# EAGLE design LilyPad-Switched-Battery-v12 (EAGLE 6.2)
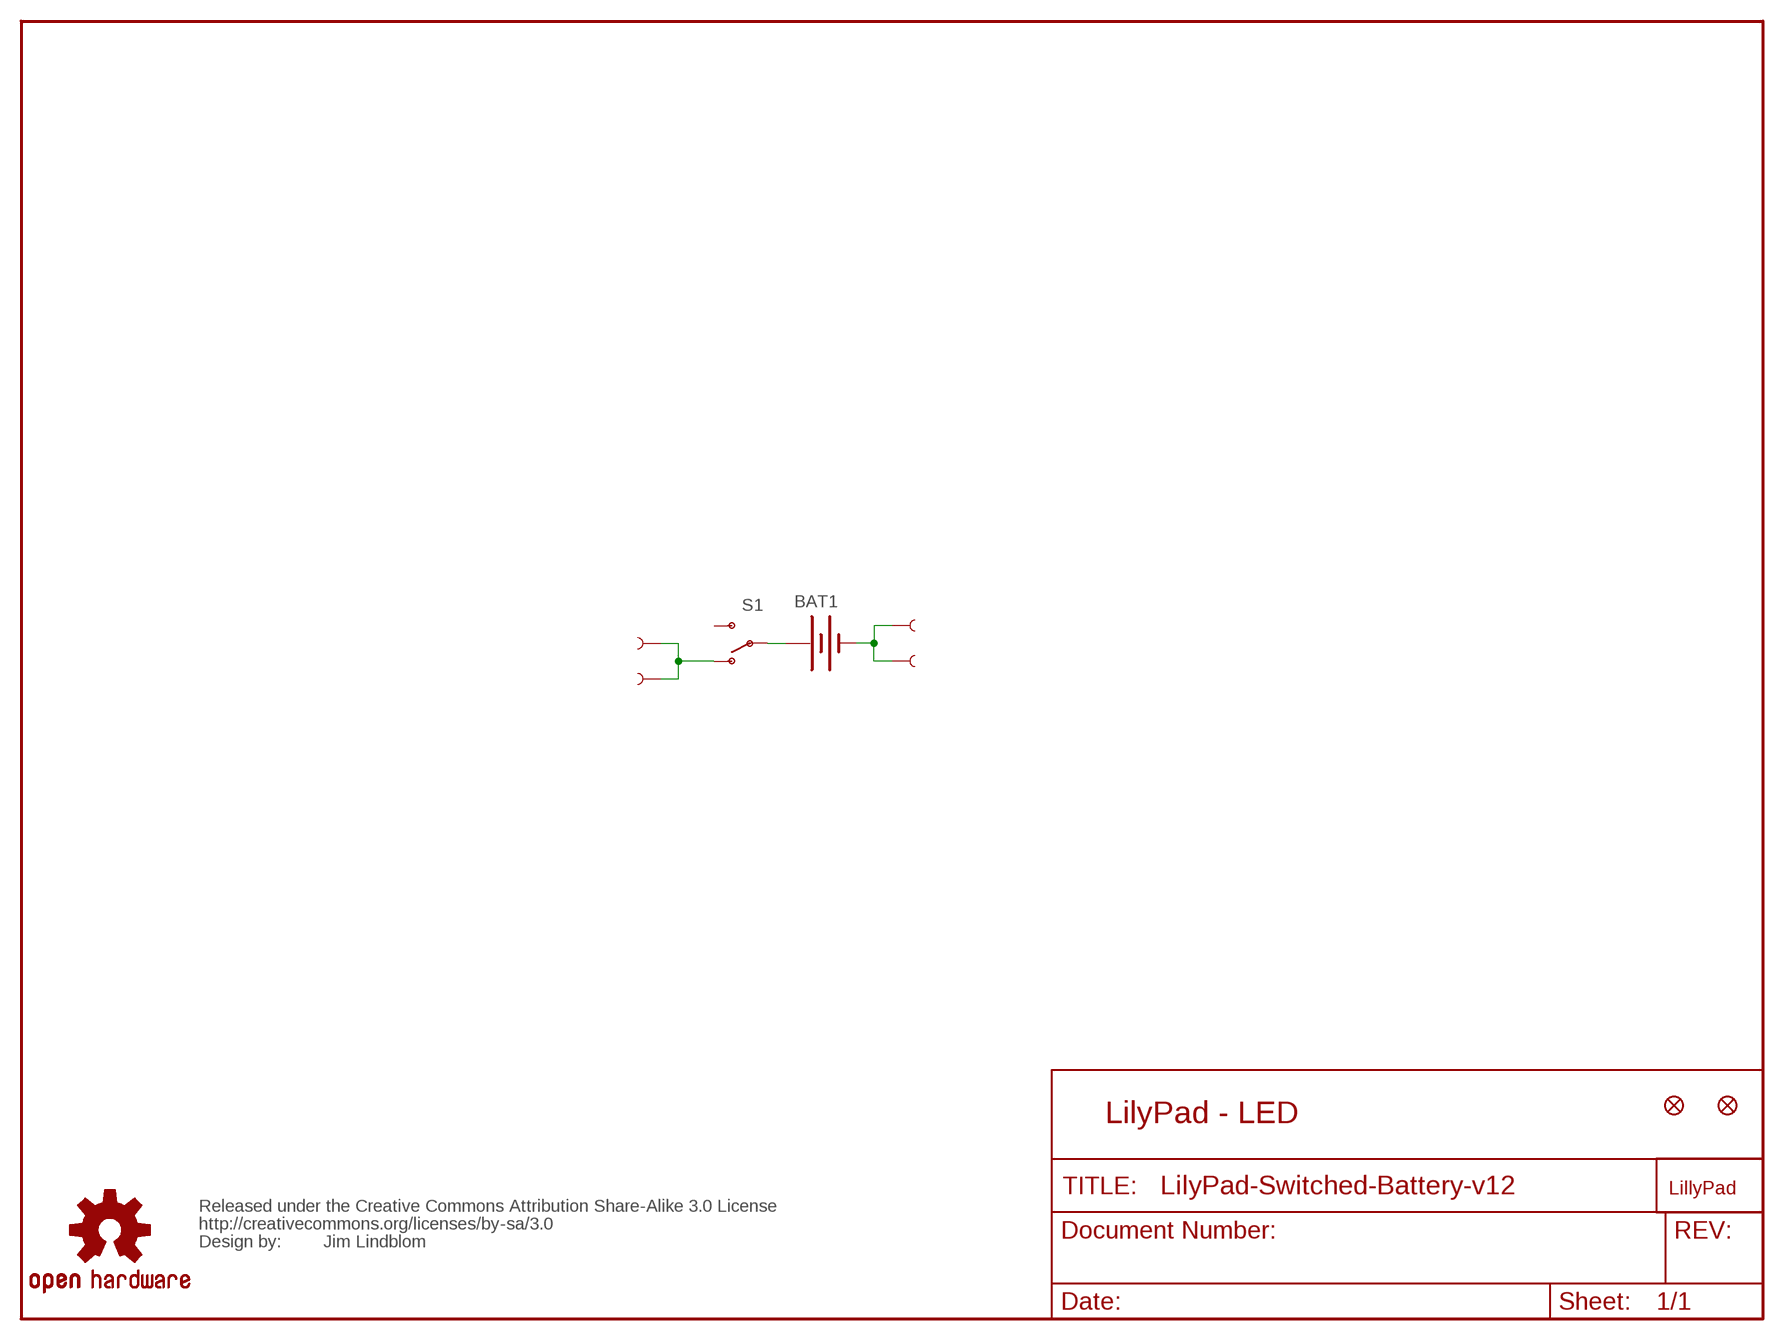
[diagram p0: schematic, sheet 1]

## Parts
BAT1  BATTERY20MM_4LEGS  [BATTCON_20MM_4LEGS]
JP1  FIDUCIALUFIDUCIAL  [MICRO-FIDUCIAL]
JP2  FIDUCIALUFIDUCIAL  [MICRO-FIDUCIAL]
S1  SWITCH-SPSTSMD  [AYZ0202]
U$1  SEWTAP6  [PETAL-SMALL-2SIDE]
U$2  SEWTAP6  [PETAL-SMALL-2SIDE]
U$3  SEWTAP6  [PETAL-SMALL-2SIDE]
U$4  SEWTAP6  [PETAL-SMALL-2SIDE]
U$5  LOGO-LPLP  [LOGO-LILYPAD]
U$7  OSHW-LOGOS  [OSHW-LOGO-S]
U$8  CREATIVE_COMMONS  [CREATIVE_COMMONS]

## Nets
N$1: S1.1(O) U$2.1 U$4.1
N$2: BAT1.2(-) U$1.1 U$3.1
N$3: BAT1.1(+) BAT1.3(+) BAT1.P$1(+) BAT1.P$2(+) S1.2(P)
Unconnected: S1.3(S)

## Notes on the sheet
- LilyPad - LED
- Jim Lindblom

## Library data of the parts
BAT1 = SparkFun-Electromechanical:BATTERY: Battery Holders
JP1 JP2 = SparkFun:FIDUCIAL: Fiducial Alignment Points
S1 = SparkFun:SWITCH-SPST: SPST Switch Simple slide switch. Spark Fun Electronics SKU : COM-00102
U$1-U$4 = LilyPad-Wearables:SEWTAP
U$5 = LilyPad-Wearables:LOGO-LP
U$7 = SparkFun-Aesthetics:OSHW-LOGO: Open Source Hardware Logo This logo indicates the piece of hardware it is found on incorporates a OSHW license and/or adheres to the definition of open source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
U$8 = SparkFun-Aesthetics:CREATIVE_COMMONS: Creative Commons License summary

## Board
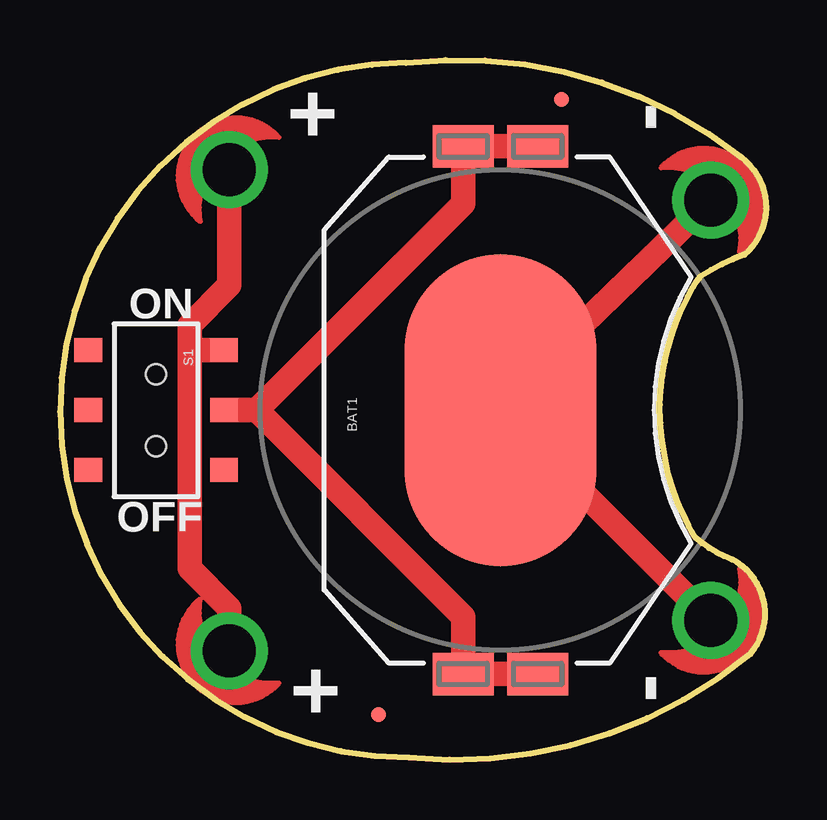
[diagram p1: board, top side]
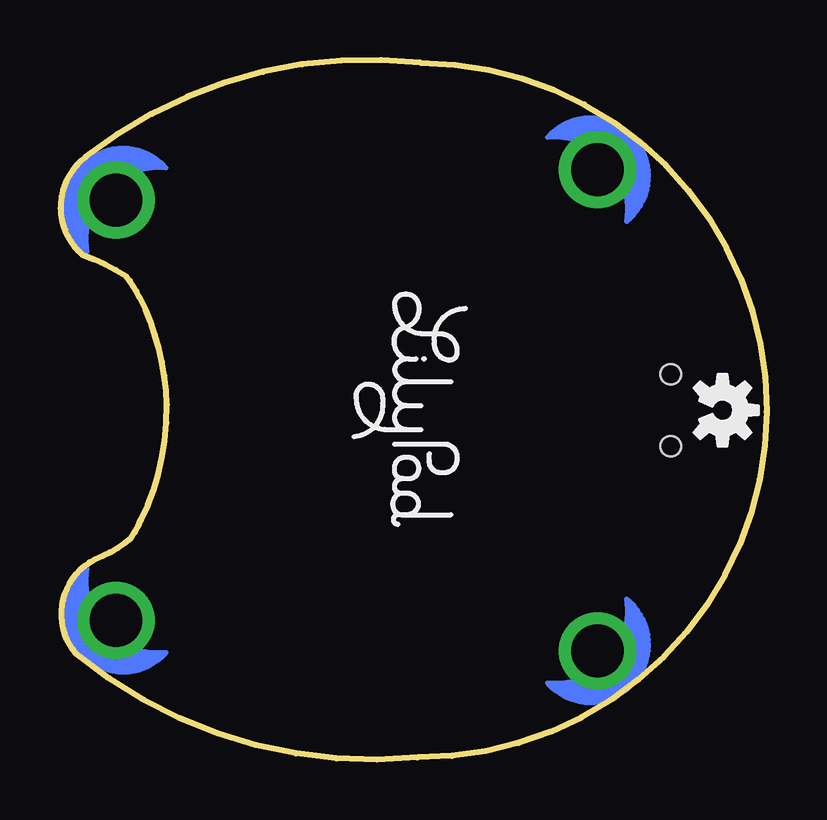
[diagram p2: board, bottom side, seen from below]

Size 29.42 x 29.17 mm. Coordinates in mm from the lower left corner, seen from the top.
Outline: 14.54,0.09 arc45 28.77,4.41 arc103 28,8.35 arc-20 26.48,9.25 arc-11 26.07,9.99 arc-17 25.21,12.55 arc-11 24.99,14.8 arc-13 25.34,17.17 arc-9 25.88,18.76 26.15,19.29 arc-14 26.7,20.16 arc-13 28.51,21.05 arc102 28.38,25.11 arc45 14.41,29.05 arc180 14.54,0.09
Copper layers (1*16): Top 0.035mm / dielectric 1.5mm / Bottom 0.035mm
Design rules: minimum track width 8mil, minimum drill 20mil, track to track 8mil, track to pad 8mil, pad to pad 8mil, via to via 8mil, smd to smd 8mil, copper to edge 8mil, drill to drill 8mil, minimum pad ring 12mil, minimum via ring 10mil, stop-mask expansion 4mil, vias tented up to drill 20mil, thermal gap 10mil

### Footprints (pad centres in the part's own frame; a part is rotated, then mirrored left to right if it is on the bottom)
BATTCON_20MM_4LEGS = smd 1.778 x 2.54: 1 -11,1.55; 3 11,1.55; P$1 -11,-1.55; P$2 11,-1.55 | smd 13 x 8: 2 0,0
MICRO-FIDUCIAL = smd 0.635 x 0.635: 1 0,0
AYZ0202 = smd 1 x 1.15: 1 -2.5,2.825; 2 0,2.825; 3 2.5,2.825; 4 -2.5,-2.825; 5 0,-2.825; 6 2.5,-2.825 | hole 0.85: 1.5,0; -1.5,0
PETAL-SMALL-2SIDE = drill 2.2: 1 0,0

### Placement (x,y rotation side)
BAT1  18.35,14.57 90 top
JP1  13.27,1.87 0 top
JP2  20.89,27.52 0 top
S1  4,14.57 270 top
U$1  27.11,5.81 47 top
U$2  7.05,4.54 313 top
U$3  27.11,23.33 133 top
U$4  7.05,24.6 227 top
U$5  14.54,14.57 270 bottom
U$7  1.84,14.57 270 bottom
U$8  not placed on the board

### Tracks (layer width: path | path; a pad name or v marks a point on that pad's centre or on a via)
N$1
  Top 1.016: U$4.1 7.05,19.78 5.4,18.13 5.4,17.11 | 5.4,17.11 5.4,7.97 7.05,6.32 U$2.1 | S1.1 5.44,17.07 5.4,17.11
N$2
  Top 1.016: 28,4.92 U$1.1 BAT1.2 18.35,14.82 U$3.1
N$3
  Top 1.016: S1.2 8.19,14.57 | 8.19,14.57 16.8,5.96 BAT1.1 BAT1.P$1 | BAT1.P$2 BAT1.3 16.8,23.18 8.19,14.57

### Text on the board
tPlace: - | + | ON | OFF | + | -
